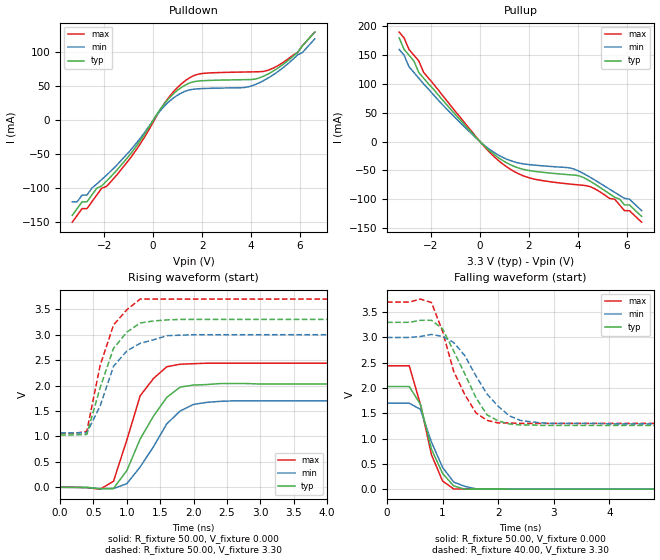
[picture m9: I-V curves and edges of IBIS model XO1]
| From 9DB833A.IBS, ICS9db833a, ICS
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|   Model XO1
[Model]   XO1
Model_type   Output
Polarity   Non-Inverting
Vmeas =   1.50V
Cref =  30.00pF
Rref =  0.000
Vref =   1.50V
C_comp   3.40pF   2.85pF   3.95pF
[Temperature Range]   25.00   70.00   0.000
[Voltage Range]   3.30V   3.00V   3.70V
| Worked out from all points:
|   slope of the pulldown table from 0 to 0.495 V, typ, clamps not added: 19 ohm
|   slope of the pullup table from 0 to 0.495 V, typ, clamps not added: 25.1 ohm
|   rising waveform, R_fixture 50.00, V_fixture 0.000: 20-80 % time 497ps typ, 524ps min, 399ps max; typ from 0 V to 2.03 V
|   rising waveform, R_fixture 50.00, V_fixture 3.30: 20-80 % time 376ps typ, 410ps min, 320ps max; typ from 1.03 V to 3.3 V
|   falling waveform, R_fixture 50.00, V_fixture 0.000: 20-80 % time 347ps typ, 394ps min, 345ps max; typ from 2.03 V to 0 V
|   falling waveform, R_fixture 40.00, V_fixture 3.30: 20-80 % time 557ps typ, 622ps min, 485ps max; typ from 3.3 V to 1.26 V
[Pulldown]
| voltage   I(typ)   I(min)   I(max)
-3.3V     -140mA     -120mA     -150mA
-3.1V     -130mA     -120mA     -140mA
-2.9V     -120mA     -110mA     -130mA
-2.7V     -120mA     -110mA     -130mA
-1V       -52.95mA   -47.18mA   -58.91mA
400mV     21.73mA    18.6mA     21.64mA
1.3V      51.77mA    42.67mA    57.97mA
2V        58.31mA    46.77mA    68.97mA
3.7V      59.9mA     48.29mA    71.19mA
4.5V      64.8mA     58.32mA    72.05mA
5.9V      100mA      96.41mA    100mA
6.6V      130mA      120mA      130mA
[Pullup]
| voltage   I(typ)   I(min)   I(max)
-3.3V     180mA      160mA      190mA
-2.5V     120mA      110mA      140mA
-2.3V     110mA      100mA      120mA
-300mV    13.74mA    11.85mA    15.55mA
900mV     -32.22mA   -26.84mA   -37.96mA
2V        -50.27mA   -39.98mA   -62.88mA
3.9V      -58.53mA   -48.83mA   -74.78mA
4.5V      -68.84mA   -62.06mA   -78.33mA
5.5V      -96.7mA    -88.18mA   -100mA
5.9V      -110mA     -98.65mA   -120mA
6.1V      -110mA     -100mA     -120mA
6.6V      -130mA     -120mA     -140mA
[Ramp]
| variable   typ   min   max
dV/dt_r   1.22/0.43n   1.02/0.52n   1.46/0.35n
dV/dt_f   1.36/0.45n   1.16/0.55n   0.63/0.17n
R_load = 50.00
[Rising Waveform]
R_fixture = 50.00
V_fixture = 0.000
V_fixture_min = 0.000
V_fixture_max = 0.000
| time   V(typ)   V(min)   V(max)
0s        370uV      2.27mV     490uV
600ps     -29.24mV   -24.48mV   -35.58mV
800ps     -22.14mV   -23.56mV   120mV
1ns       330mV      72.36mV    930mV
1.2ns     950mV      400mV      1.8V
1.6ns     1.77V      1.25V      2.37V
1.8ns     1.97V      1.5V       2.42V
2ns       2.01V      1.63V      2.43V
2.6ns     2.04V      1.7V       2.44V
10ns      2.03V      1.7V       2.44V
[Rising Waveform]
R_fixture = 50.00
V_fixture = 3.30
V_fixture_min = 3.00
V_fixture_max = 3.70
| time   V(typ)   V(min)   V(max)
0s        1.03V      1.07V      1.06V
200ps     1.03V      1.07V      1.06V
400ps     1.04V      1.07V      1.1V
600ps     1.96V      1.6V       2.4V
800ps     2.73V      2.38V      3.19V
1ns       3.05V      2.68V      3.49V
1.2ns     3.23V      2.83V      3.7V
1.6ns     3.29V      2.98V      3.7V
2ns       3.3V       3V         3.7V
10ns      3.3V       3V         3.7V
[Falling Waveform]
R_fixture = 50.00
V_fixture = 0.000
V_fixture_min = 0.000
V_fixture_max = 0.000
| time   V(typ)   V(min)   V(max)
0s        2.03V      1.7V       2.44V
400ps     2.03V      1.7V       2.44V
600ps     1.68V      1.58V      1.68V
800ps     790mV      930mV      680mV
1ns       310mV      430mV      160mV
1.2ns     63.37mV    140mV      3.92mV
1.4ns     -120uV     54.71mV    3.64mV
1.6ns     2.17mV     7.6mV      2.28mV
1.8ns     2.07mV     1.7mV      1.4mV
10ns      370uV      300uV      490uV
[Falling Waveform]
R_fixture = 40.00
V_fixture = 3.30
V_fixture_min = 3.00
V_fixture_max = 3.70
| time   V(typ)   V(min)   V(max)
0s        3.3V       3V         3.7V
800ps     3.34V      3.06V      3.69V
1ns       3.17V      3.02V      3.12V
1.2ns     2.73V      2.9V       2.33V
1.4ns     2.28V      2.64V      1.87V
1.8ns     1.47V      1.88V      1.36V
2ns       1.35V      1.64V      1.31V
2.4ns     1.27V      1.36V      1.3V
3ns       1.26V      1.3V       1.3V
10ns      1.26V      1.29V      1.3V
